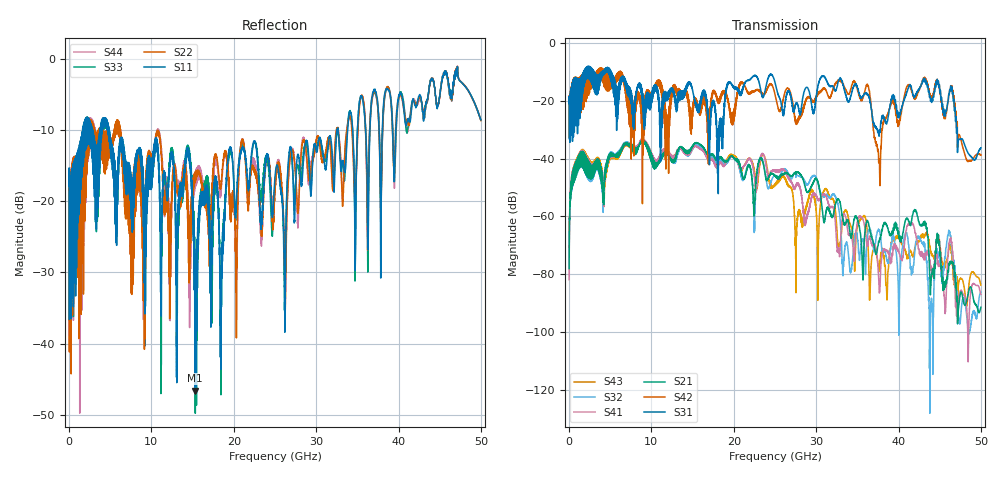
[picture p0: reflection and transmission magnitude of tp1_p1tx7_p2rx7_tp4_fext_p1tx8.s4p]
! 100G CR Analysis
! File: tp1_p1tx7_p2rx7_tp4_fext_p1tx8
! Description: 2m Cu Cable, OSFP, TP1-TP4
! Port Mapping
! Port1 -- P1TX8N
! Port2 -- P2RX7N
! Port3 -- P1TX8P
! Port4 -- P2RX7P
# GHz S MA R 50.00
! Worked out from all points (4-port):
!   5000 points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, 10 MHz to 50 GHz, reference 50 ohm
!   strongest paths, dB at 10 MHz, 12.51 GHz, 25.01 GHz, 37.51 GHz, 50 GHz:
!     S31: -20.6, -15.7, -13.7, -30.7, -36.3
!     S42: -20.5, -15.9, -17.8, -36.7, -38.8
!     S21: -78.1, -41.2, -45.8, -70.2, -91.5
!     S41: -81.9, -39.6, -44.4, -77.2, -87.0
!     S32: -70.9, -41.0, -45.8, -65.1, -86.2
!     S43: -70.8, -39.5, -49.2, -77.0, -83.8
!   lowest |S11| = -46.6 dB at 15.32 GHz (marker M1), VSWR 1.01, Z = 49.9 - j0.462 ohm
!   |S11| at or under -10 dB: start of sweep to 1.658 GHz; 4.861 GHz to 32.52 GHz (27.66 GHz wide, 148 % of centre); 32.66 GHz to 33.81 GHz (1.154 GHz wide, 3.47 % of centre)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
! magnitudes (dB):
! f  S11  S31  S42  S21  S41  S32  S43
! 10 MHz  -17.9  -20.6  -20.5  -78.1  -81.9  -70.9  -70.8
! 1.4 GHz  -14.2  -12.4  -11.6  -42.8  -42.2  -43.0  -41.7
! 15.32 GHz  -46.6  -21.0  -19.3  -34.7  -35.7  -35.5  -35.6
! 34.62 GHz  -16.0  -14.7  -13.4  -61.0  -75.6  -68.5  -74.8
! 37.65 GHz  -10.2  -32.2  -41.5  -68.9  -85.3  -65.0  -78.8
! 43.21 GHz  -6.9  -13.4  -12.9  -62.7  -74.3  -71.0  -66.7
! 50 GHz  -8.6  -36.3  -38.8  -91.5  -87.0  -86.2  -83.8
